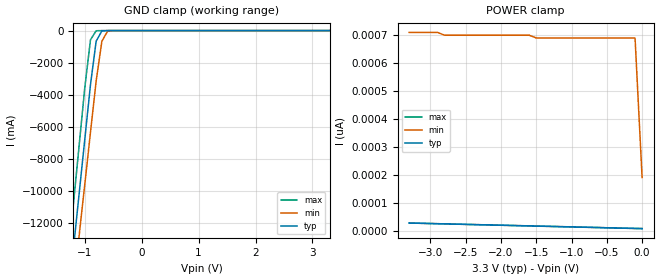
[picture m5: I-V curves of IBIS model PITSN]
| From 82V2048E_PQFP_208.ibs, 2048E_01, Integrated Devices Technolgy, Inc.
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|   Model PITSN
[Model]   PITSN
Model_type   Input
Polarity   Non-Inverting
Vinl =   0.74V
Vinh =   2.10V
C_comp   3.50pF   4.00pF   3.50pF
[Temperature Range]   25.00   85.00   -40.00
[Voltage Range]   3.30V   3.00V   3.60V
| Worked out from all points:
|   GND clamp passes 1 mA (typ) near -0.60 V on its own axis
[GND_clamp]
| voltage   I(typ)   I(min)   I(max)
-3.3V     -85.44A    -84.07A    -87.3A
-1.3V     -17.05A    -19.32A    -14.49A
-1.2V     -13.64A    -16.09A    -10.85A
-1.1V     -10.22A    -12.85A    -7.21A
-1V       -6.8A      -9.61A     -3.57A
-900mV    -3.38A     -6.37A     -580mA
-800mV    -660mA     -3.14A     -10.9mA
-700mV    -23.2mA    -670mA     -750uA
-600mV    -570uA     -41.03mA   -46.43uA
-400mV    -420nA     -77.43uA   -33.21nA
3.3V      6.8pA      690pA      5.81pA
[POWER_clamp]
| voltage   I(typ)   I(min)   I(max)
-3.3V     27.02pA    710pA      27pA
-2.9V     24.52pA    710pA      24.6pA
-2.8V     23.9pA     700pA      24pA
-1.6V     16.56pA    700pA      16.8pA
-1.5V     15.96pA    690pA      16.2pA
-100mV    7.48pA     690pA      7.72pA
0V        6.8pA      190pA      7.2pA
